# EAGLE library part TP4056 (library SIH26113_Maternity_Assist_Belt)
NanJing Top Power TP4056-42-SOP8-PP 1 A standalone linear Li-ion charger, 4.2 V float. Pin map from the TP4056 datasheet pin description (page 2).
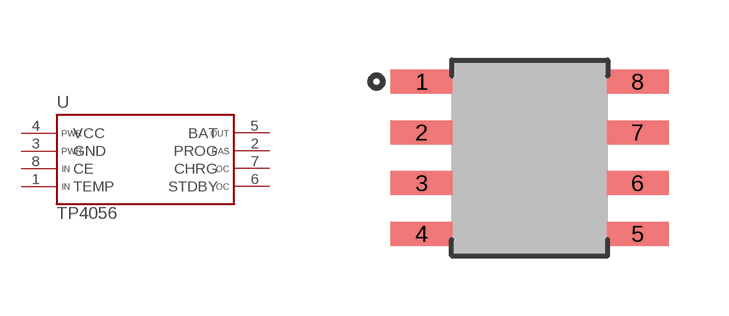
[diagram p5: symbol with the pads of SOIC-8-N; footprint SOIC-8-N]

Designator prefix U

## TP4056  [SOIC-8-N]
1  TEMP  in
2  PROG  pas
3  GND  pwr
4  VCC  pwr
5  BAT  out
6  STDBY  oc
7  CHRG  oc
8  CE  in

## Footprint SOIC-8-N (pad centres in mm)
SOIC-8 narrow (150 mil body). Body 4.90 x 3.90 mm, lead span 6.00 mm, 1.27 mm pitch. Lands 1.55 x 0.60 mm at 5.40 mm span (IPC-7351B SOIC127P600X175-8N Nominal).
smd 1.55 x 0.6: 1 -2.7,1.905; 2 -2.7,0.635; 3 -2.7,-0.635; 4 -2.7,-1.905; 5 2.7,-1.905; 6 2.7,-0.635; 7 2.7,0.635; 8 2.7,1.905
